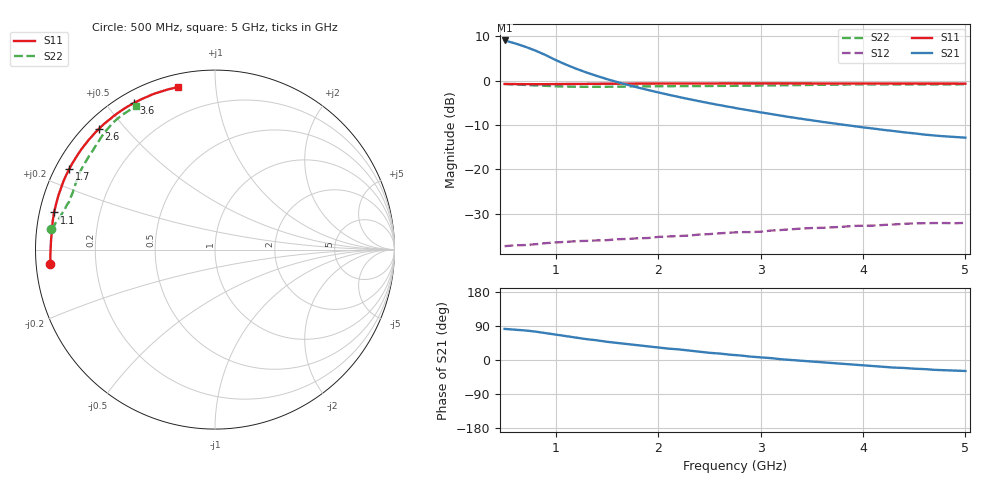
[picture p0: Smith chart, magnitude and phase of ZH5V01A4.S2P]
! SIEMENS Discrete & RF Semiconductors
! CLY38
! GaAs Power FET in MWP-35
! VDS = 5 V  ID = 1400 mA
! Common Source S-Parameters:  August  1998
# GHz  S  MA  R  50
!  f  S11  S21  S12  S22
! GHz  MAG  ANG  MAG  ANG  MAG  ANG  MAG  ANG
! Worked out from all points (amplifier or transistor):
!   46 points, 500 MHz to 5 GHz, reference 50 ohm
!   highest |S21| = 9.1 dB at 500 MHz (marker M1)
!   |S21| within 3 dB of that: start of sweep to 871.2 MHz
!   unconditionally stable (mu >= 1): 1.006 GHz to end of sweep
!   at 1.2 GHz: K = 1.20, MAG = 16.8 dB, |S12| = -36.2 dB
!   at 2.8 GHz: K = 1.86, MAG = 8.6 dB, |S12| = -34.2 dB
!   at 5 GHz: K = 2.34, MAG = 3.1 dB, |S12| = -32.1 dB
!   S11 on the Smith chart (normalised r, x): 500 MHz: 0.04, -0.04; 1.1 GHz: 0.04, +0.11; 1.7 GHz: 0.04, +0.26; 2.6 GHz: 0.04, +0.42; 3.6 GHz: 0.05, +0.59; 5 GHz: 0.06, +0.79
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0.5  0.921 -175.0  2.85 82.0  0.0136 19.0  0.919 173.0
0.7  0.916 180.0  2.424 78.0  0.014 18.0  0.898 170.0
0.9  0.915 173.0  1.951 71.0  0.0147 15.0  0.877 167.0
1  0.918 170.0  1.71 67.0  0.015 14.0  0.867 165.0
1.1  0.92 167.0  1.52 63.0  0.0152 14.0  0.861 163.0
1.2  0.921 164.0  1.366 59.0  0.0155 14.0  0.856 162.0
1.3  0.923 161.0  1.239 55.0  0.0156 14.0  0.855 160.0
1.5  0.926 156.0  1.044 48.0  0.0159 14.0  0.856 157.0
1.7  0.928 151.0  0.9 42.0  0.0164 14.0  0.861 154.0
2  0.93 145.0  0.739 33.0  0.0173 14.0  0.867 150.0
2.4  0.932 137.0  0.588 22.0  0.0184 13.0  0.872 145.0
2.6  0.933 134.0  0.531 17.0  0.019 13.0  0.875 143.0
2.8  0.934 131.0  0.482 12.0  0.0196 12.0  0.879 140.0
3.2  0.934 124.0  0.404 2.0  0.0207 10.0  0.889 136.0
3.5  0.933 120.0  0.358 -4.0  0.0218 8.0  0.898 133.0
3.6  0.933 119.0  0.344 -6.0  0.0219 7.0  0.901 131.0
4  0.932 113.0  0.298 -14.0  0.0231 6.0  0.909 127.0
4.3  0.931 110.0  0.271 -20.0  0.0239 5.0  0.911 125.0
4.4  0.93 108.0  0.262 -21.0  0.0243 5.0  0.911 124.0
4.8  0.929 104.0  0.236 -27.0  0.0248 3.0  0.912 120.0
4.9  0.929 103.0  0.232 -28.0  0.0247 3.0  0.912 120.0
5  0.928 103.0  0.228 -29.0  0.0249 2.0  0.913 119.0
